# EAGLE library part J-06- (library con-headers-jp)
HEADER JACK PINS
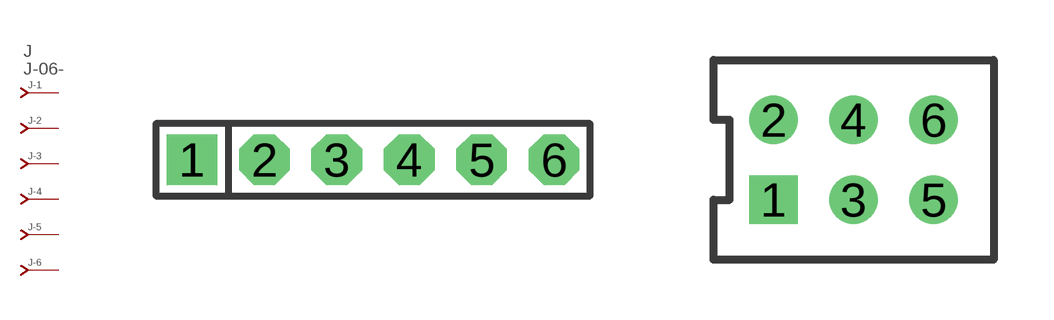
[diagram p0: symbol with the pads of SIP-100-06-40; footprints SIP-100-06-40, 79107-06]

Designator prefix J; gates -2=J-N -3=J-N -4=J-N -5=J-N -6=J-N -1=J-NV

## J-06-SIP-100-40  [SIP-100-06-40]
1  -1:J  pas
2  -2:J  pas
3  -3:J  pas
4  -4:J  pas
5  -5:J  pas
6  -6:J  pas

## J-06-79107  [79107-06]
Pads as for SIP-100-06-40

## J-06-79109  [79109-06]
Pads as for SIP-100-06-40

## J-06-87340  [87340-06]
Pads as for SIP-100-06-40

## J-06-535512  [535512-06]
Pads as for SIP-100-06-40

## J-06-100-2X03  [DIL-100-2X03]
Pads as for SIP-100-06-40

## J-06-100-2X03_M  [DIL-100-2X03_M]
Pads as for SIP-100-06-40

## J-06-2MM-2X03  [DIL-2MM-2X03]
Pads as for SIP-100-06-40

## J-06-2MM-2X03_M  [DIL-2MM-2X03_M]
Pads as for SIP-100-06-40

## J-06-SIP-100-32  [SIP-100-06-32]
Pads as for SIP-100-06-40

## J-06-SIP-100-40Y  [SIP-100-06-40Y]
Pads as for SIP-100-06-40

## J-06-SIP-100-32Y  [SIP-100-06-32Y]
Pads as for SIP-100-06-40

## J-06-KK-4455-B06  [KK-4455-B06]
Pads as for SIP-100-06-40

## J-06-KK-4455-A06  [KK-4455-A06]
Pads as for SIP-100-06-40

## J-06-KK-4455-C06  [KK-4455-C06]
Pads as for SIP-100-06-40

## Footprint SIP-100-06-40 (pad centres in mm)
SIP Header - 0.1", 40 mil drill
drill 1.016 pad 1.778 square: 1 -6.35,0
drill 1.016 pad 1.778 octagon: 2 -3.81,0; 3 -1.27,0; 4 1.27,0; 5 3.81,0; 6 6.35,0

## Footprint 79107-06 (pad centres in mm)
Molex Board-To-Board Receptacal 2.00mm (.079") Pitch Milli-Grid Header, Vertical, Through-Hole Mates with: 87759, 87762, 87758, 87760
drill 0.711 square: 1 -2,-1
drill 0.711: 2 -2,1; 3 0,-1; 4 0,1; 5 2,-1; 6 2,1

## Footprint 79109-06 (pad centres in mm)
Molex Board-to-Board Receptacal 2.00mm (.079") Pitch Milli-Grid Header, Vertical, Top/Bottom Entry Mates with: 87758, 87759, 87760, 87831, 87832, 87833
smd 1.12 x 1.83: 1 -2,-2.65; 2 -2,2.65; 3 0,-2.65; 4 0,2.65; 5 2,-2.65; 6 2,2.65
hole 0.914 at -1,0
hole 0.914 at -2,1
hole 0.914 at -2,-1
hole 0.914 at 0,-1
hole 0.914 at 0,1
hole 0.914 at 2,-1
hole 0.914 at 2,1
hole 0.914 at 1,0

## Footprint 87340-06 (pad centres in mm)
Molex Board-To-Board Receptacal 2.00mm (.079") Pitch Milli-Grid Header, Vertical, Top/Bottom Entry Mates with: 87758, 87759, 87760, 87831, 87832, 87833
smd 1 x 1.75: 1 -2,-2.5; 2 -2,2.5; 3 0,-2.5; 4 0,2.5; 5 2,-2.5; 6 2,2.5
hole 0.914 at -3,0
hole 0.914 at -2,1
hole 0.914 at -2,-1
hole 0.914 at 0,-1
hole 0.914 at 0,1
hole 0.914 at 3,0
hole 0.914 at 2,1
hole 0.914 at 2,-1

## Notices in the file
Copyright (C) 2008, Bob Starr
